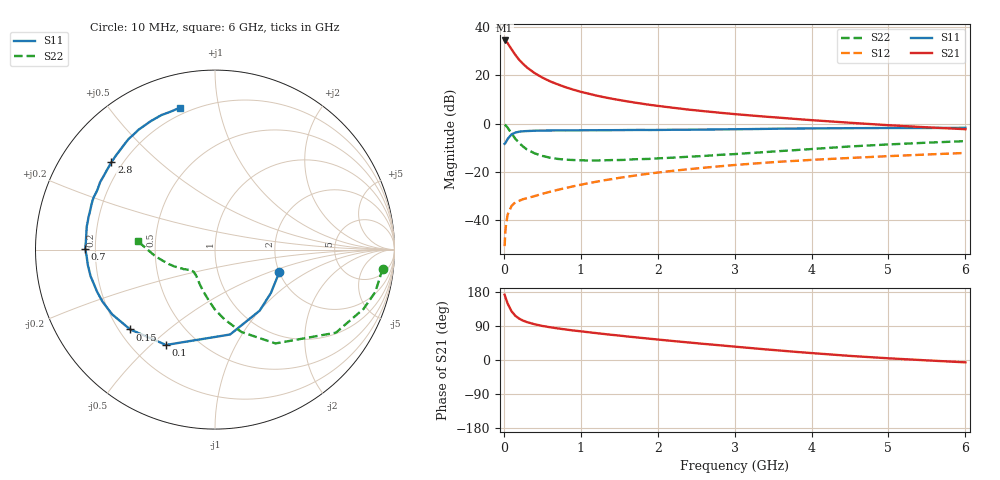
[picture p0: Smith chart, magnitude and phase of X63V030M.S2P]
! SIEMENS Small Signal Semiconductors
! BFP193W
! Si NPN RF Bipolar Junction Transistor in SOT343
! VCE = 3 V  IC = 30 mA
! Common Emitter S-Parameters:  April 1994
# GHz  S  MA  R  50
!  f  S11  S21  S12  S22
! GHz  MAG  ANG  MAG  ANG  MAG  ANG  MAG  ANG
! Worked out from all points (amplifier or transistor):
!   40 points, 10 MHz to 6 GHz, reference 50 ohm
!   highest |S21| = 34.4 dB at 10 MHz (marker M1)
!   |S21| within 3 dB of that: start of sweep to 87.27 MHz
!   unconditionally stable (mu >= 1): 784.3 MHz to 3.971 GHz
!   at 200 MHz: K = 0.45, MSG = 29.2 dB, |S12| = -32.0 dB
!   at 1.5 GHz: K = 1.12, MAG = 14.0 dB, |S12| = -22.5 dB
!   at 6 GHz: K = 0.94, MSG = 4.9 dB, |S12| = -12.2 dB
!   lowest NFmin = 1.90 dB at 450 MHz
!   S11 on the Smith chart (normalised r, x): 10 MHz: 2.00, -0.58; 100 MHz: 0.34, -0.56; 150 MHz: 0.24, -0.38; 700 MHz: 0.16, +0.00; 2.8 GHz: 0.16, +0.36; 6 GHz: 0.16, +0.77
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0.01  0.3797 -19.2  52.23 172.3  0.0029 84.0  0.94 -6.5
0.02  0.3942 -37.8  51.52 166.3  0.0059 74.5  0.924 -14.8
0.03  0.4215 -53.8  50 160.1  0.0085 75.0  0.8914 -21.7
0.05  0.4804 -79.9  45.63 148.6  0.0131 65.1  0.8173 -34.5
0.1  0.5974 -117.2  34.41 128.7  0.0197 49.7  0.622 -57.2
0.15  0.649 -136.7  26.22 116.5  0.0235 43.8  0.4823 -72.2
0.2  0.6772 -147.8  20.73 109.1  0.0252 41.8  0.3919 -82.3
0.25  0.6909 -155.3  17.14 103.9  0.0272 42.0  0.3345 -90.0
0.3  0.6975 -160.3  14.45 100.1  0.0285 42.2  0.2905 -96.2
0.4  0.709 -168.0  11.04 94.3  0.0315 44.7  0.2416 -105.6
0.5  0.7138 -173.1  8.924 89.9  0.0351 47.9  0.2138 -112.9
0.6  0.7162 -177.1  7.461 86.4  0.0387 49.8  0.1962 -118.5
0.7  0.7231 179.6  6.46 83.4  0.0424 52.0  0.1852 -122.7
0.9  0.7215 174.1  5.031 78.0  0.0501 54.8  0.1756 -129.1
1.1  0.7261 169.7  4.145 73.3  0.0582 56.9  0.1717 -133.5
1.6  0.7328 159.9  2.879 62.2  0.0793 58.1  0.1775 -139.7
2.2  0.7421 149.6  2.116 50.1  0.105 56.5  0.1966 -146.3
2.8  0.7547 139.9  1.675 39.0  0.1301 53.3  0.2243 -152.4
3.2  0.7659 133.8  1.472 31.7  0.1464 50.7  0.2451 -157.4
4.5  0.8001 116.7  1.036 10.8  0.1938 41.7  0.3349 -173.7
5.5  0.8071 108.1  0.834 -1.0  0.2285 35.2  0.4011 177.0
6  0.8145 103.8  0.763 -6.2  0.246 32.3  0.4319 173.6
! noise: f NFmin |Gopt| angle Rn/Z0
0.45  1.9  0.4  180  0.09
0.9  1.95  0.43  -173  0.11
1.8  2.4  0.58  -144  0.24
